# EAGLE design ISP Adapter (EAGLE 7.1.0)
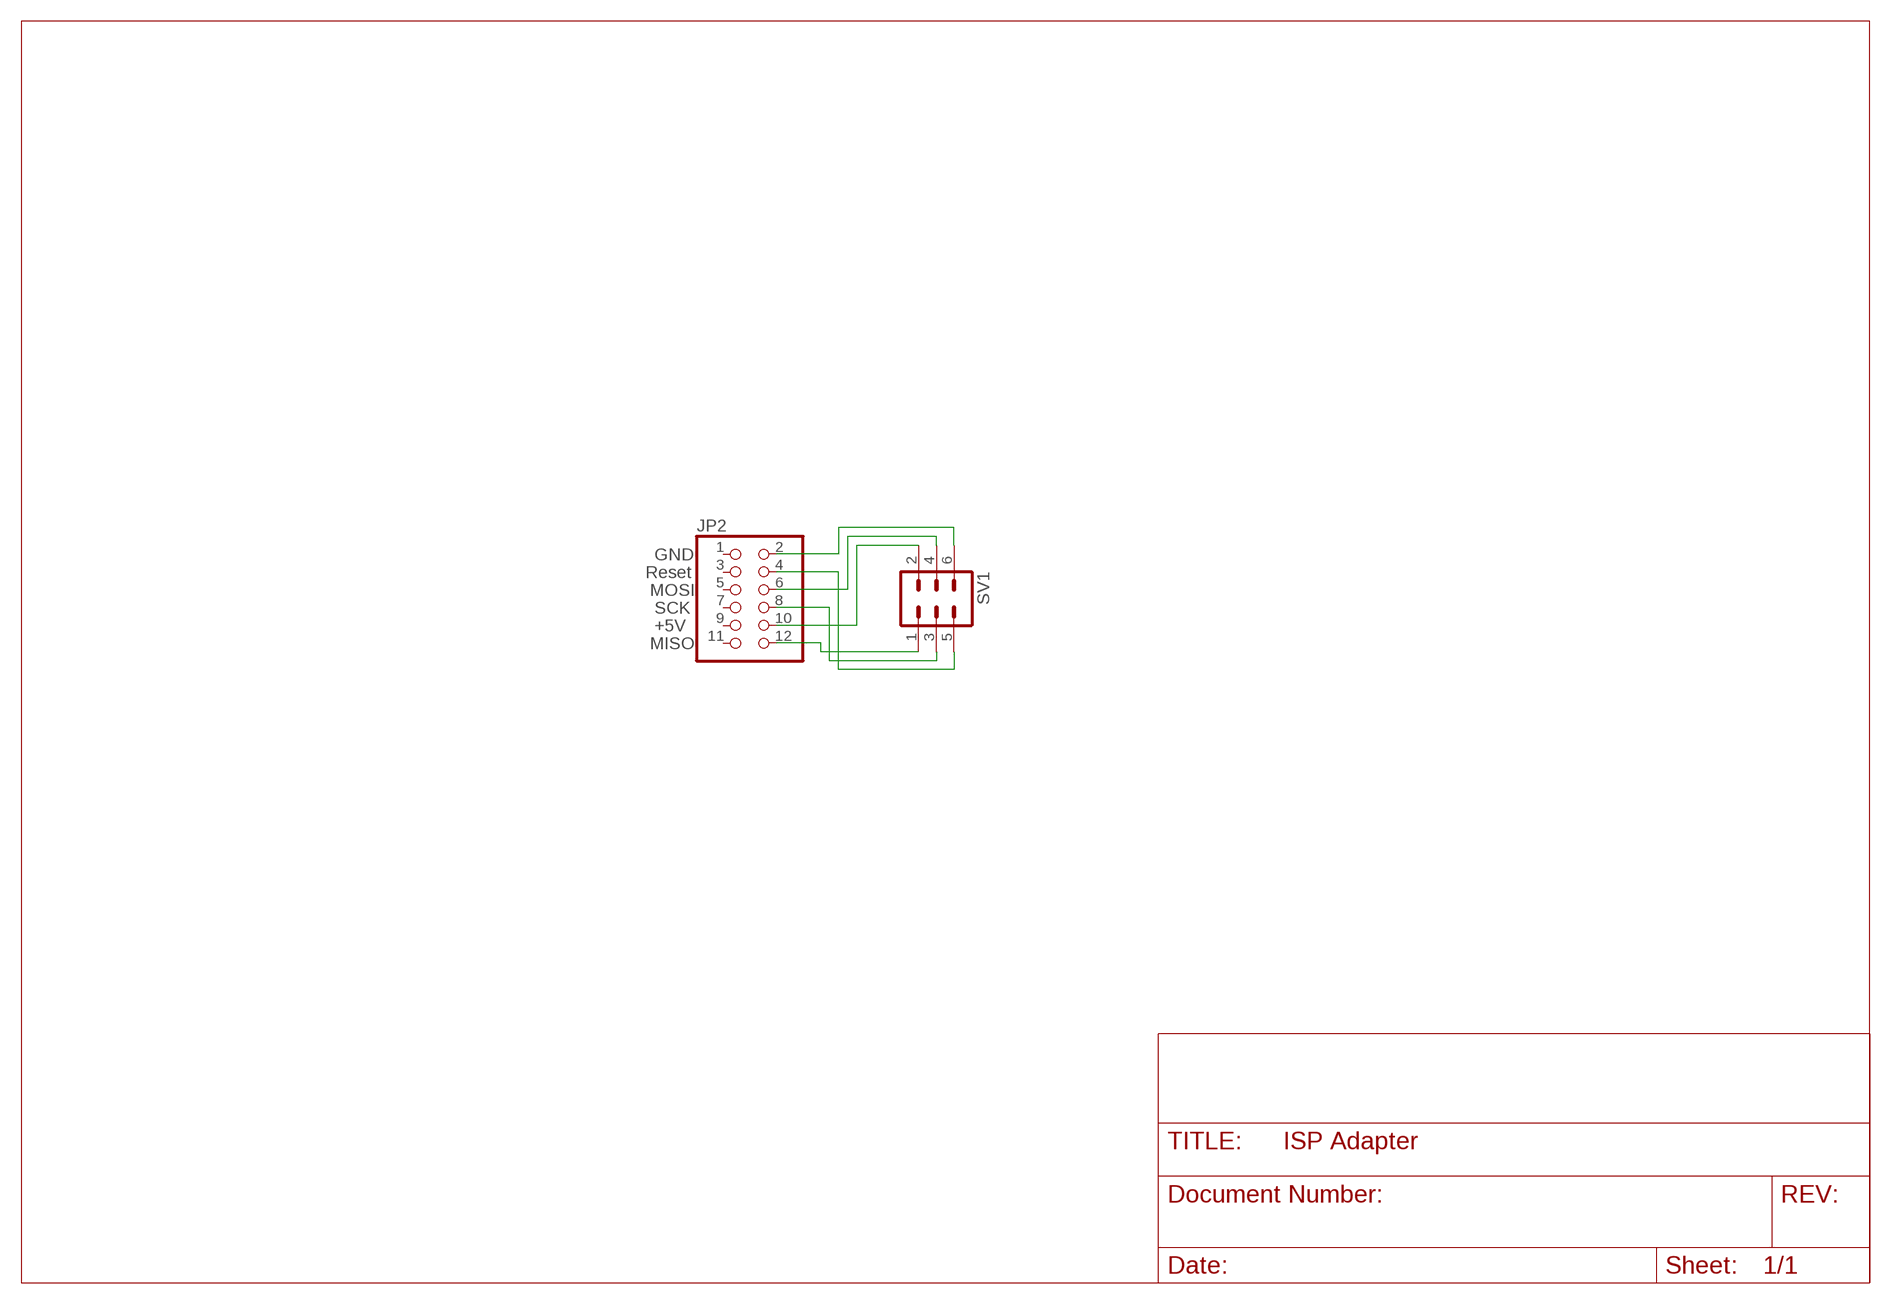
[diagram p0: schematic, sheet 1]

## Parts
JP2  PINHD-2X6  [2X06]
SV1  ML6  [ML6]

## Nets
N$1: JP2.12 SV1.1
N$2: JP2.8 SV1.3
N$3: JP2.4 SV1.5
N$4: JP2.10 SV1.2
N$5: JP2.6 SV1.4
N$6: JP2.2 SV1.6
Unconnected: JP2.1 JP2.3 JP2.5 JP2.7 JP2.9 JP2.11

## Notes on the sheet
- GND
- Reset
- MOSI
- SCK
- +5V
- MISO

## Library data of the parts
JP2 = pinhead:PINHD-2X6: PIN HEADER
SV1 = con-harting-ml:ML6: HARTING

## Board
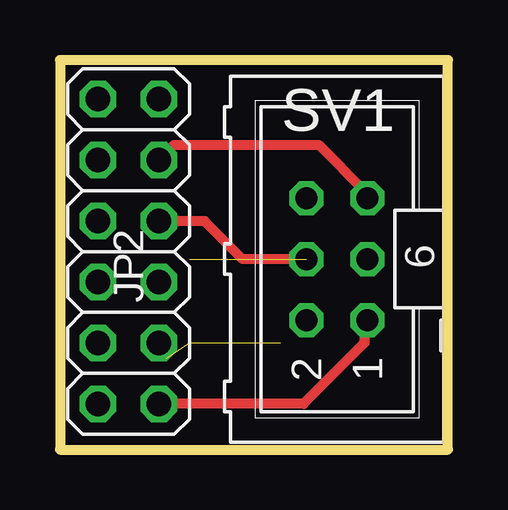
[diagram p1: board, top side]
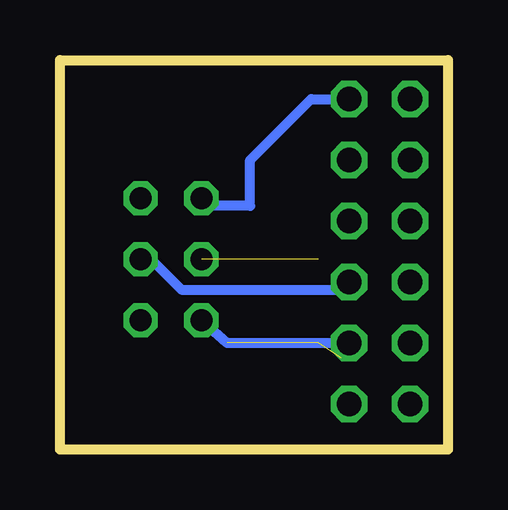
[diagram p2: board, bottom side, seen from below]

Size 16.18 x 16.23 mm. Coordinates in mm from the lower left corner, seen from the top.
Outline: 0,0 16.18,0 16.18,16.23 0,16.23 0,0
Copper layers (1*16): Top 0.035mm / dielectric 1.5mm / Bottom 0.035mm
Design rules "default": minimum track width 10mil, minimum drill 24mil, track to track 8mil, track to pad 8mil, pad to pad 8mil, via to via 8mil, smd to smd 8mil, copper to edge 40mil, drill to drill 8mil, minimum pad ring 10mil, minimum via ring 8mil, stop-mask expansion 4mil, vias tented up to drill 0mil, thermal gap 10mil

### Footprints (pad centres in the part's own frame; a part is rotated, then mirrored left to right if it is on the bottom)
2X06 = drill 1.016 octagon: 1 -6.35,-1.27; 2 -6.35,1.27; 3 -3.81,-1.27; 4 -3.81,1.27; 5 -1.27,-1.27; 6 -1.27,1.27; 7 1.27,-1.27; 8 1.27,1.27; 9 3.81,-1.27; 10 3.81,1.27; 11 6.35,-1.27; 12 6.35,1.27
ML6 = drill 0.914 octagon: 1 -2.54,-1.27; 2 -2.54,1.27; 3 0,-1.27; 4 0,1.27; 5 2.54,-1.27; 6 2.54,1.27

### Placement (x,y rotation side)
JP2  2.86,8.26 270 top
SV1  11.56,7.94 90 top

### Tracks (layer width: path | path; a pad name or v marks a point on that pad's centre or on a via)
N$1
  Top 0.406: SV1.1 12.7,4.45 10.16,1.91 JP2.12
N$2
  Bottom 0.406: SV1.3 12.38,7.94 11.11,6.67 4.45,6.67 JP2.8
N$3
  Top 0.406: SV1.5 12.7,10.79 10.79,12.7 4.76,12.7 JP2.4
N$4  (2 unrouted)
  Bottom 0.406: SV1.2 9.21,4.45 JP2.10
N$5  (1 unrouted)
  Top 0.406: 10.48,7.94 SV1.4 7.62,7.94 6.03,9.53 JP2.6
N$6
  Bottom 0.406: SV1.6 10.16,10.16 8.26,10.16 8.26,12.06 5.71,14.61 JP2.2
